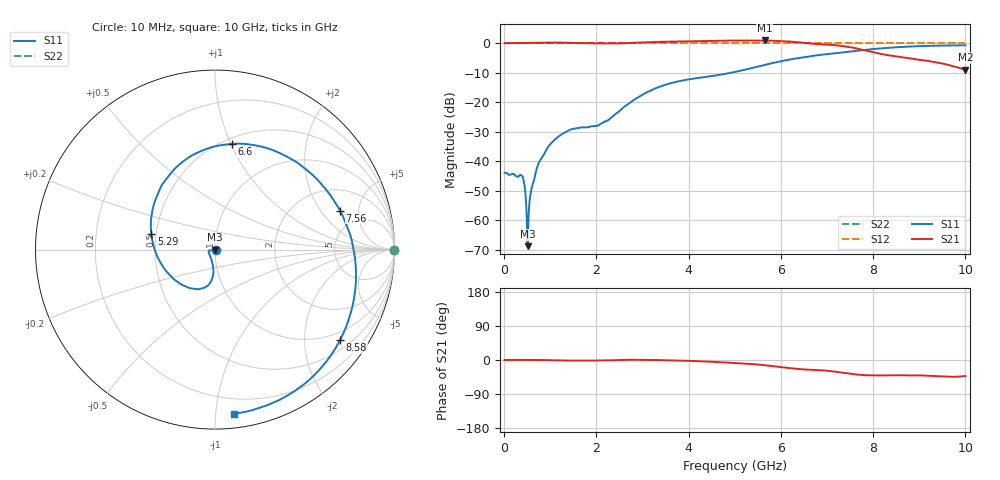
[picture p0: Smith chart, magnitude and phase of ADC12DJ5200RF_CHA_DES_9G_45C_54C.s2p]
! Texas Instruments, Inc.
! ADC12DJ5200RF - CH A S-Parameters (DES Mode, Fs = 9 GSPS, 45 degC case, 54 degC juntion)
! Port 1 represents the 100-ohm differenal input, Port 2 the digital output
! freq  dbS11  angS11  dbS21 angS21 dbS12 angS12 dbS22 angS22
# HZ S DB R 100
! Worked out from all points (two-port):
!   1000 points, 10 MHz to 10 GHz, reference 100 ohm
!   highest |S21| = 0.93 dB at 5.65 GHz (marker M1); lowest = -8.9 dB at 10 GHz (marker M2)
!   |S21| within 3 dB of the highest: start of sweep to 7.724 GHz
!   lowest |S11| = -68.9 dB at 510 MHz (marker M3), VSWR 1.00, Z = 100 - j0.0713 ohm
!   |S11| at or under -10 dB: start of sweep to 4.932 GHz
!   |S22| runs from 0.0 to 0.0 dB; largest |S21 - S12| = 0.77
!   S11 on the Smith chart (normalised r, x): 10 MHz: 1.01, -0.00; 5.29 GHz: 0.47, +0.10; 6.6 GHz: 0.55, +1.01; 7.56 GHz: 3.35, +3.13; 8.58 GHz: 0.75, -2.91; 10 GHz: 0.09, -1.12
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1e7  -43.98 -7.6  0.00 0.0  0.00 0.0  0.00 0.0
3.8e8  -44.92 -10.5  0.07 0.3  0.00 0.0  0.00 0.0
4.3e8  -47.24 -0.5  0.08 0.3  0.00 0.0  0.00 0.0
4.7e8  -52.81 6.8  0.09 0.3  0.00 0.0  0.00 0.0
5.1e8  -68.87 -81.6  0.11 0.3  0.00 0.0  0.00 0.0
6e8  -48.82 -136.8  0.14 0.2  0.00 0.0  0.00 0.0
7.1e8  -42.37 -157.4  0.15 0.2  0.00 0.0  0.00 0.0
9.4e8  -35.52 -169.1  0.23 -0.3  0.00 0.0  0.00 0.0
1.26e9  -30.80 -171.7  0.20 -1.3  0.00 0.0  0.00 0.0
1.68e9  -28.56 -163.4  0.04 -1.7  0.00 0.0  0.00 0.0
2.24e9  -26.25 -119.8  -0.06 -1.0  0.00 0.0  0.00 0.0
3.34e9  -14.98 -96.9  0.46 -0.1  0.00 0.0  0.00 0.0
4.24e9  -11.72 -125.9  0.74 -3.2  0.00 0.0  0.00 0.0
5.01e9  -9.74 -174.4  0.90 -8.0  0.00 0.0  0.00 0.0
5.29e9  -8.74 165.9  0.89 -10.0  0.00 0.0  0.00 0.0
5.65e9  -7.37 141.9  0.93 -13.8  0.00 0.0  0.00 0.0
6.6e9  -4.49 81.1  -0.03 -25.5  0.00 0.0  0.00 0.0
6.67e9  -4.33 76.5  -0.15 -26.0  0.00 0.0  0.00 0.0
7.56e9  -2.73 17.4  -1.51 -37.1  0.00 0.0  0.00 0.0
8.34e9  -1.56 -25.8  -4.11 -40.5  0.00 0.0  0.00 0.0
8.58e9  -1.31 -35.9  -4.62 -40.3  0.00 0.0  0.00 0.0
1e10  -0.71 -83.2  -8.93 -42.3  0.00 0.0  0.00 0.0
